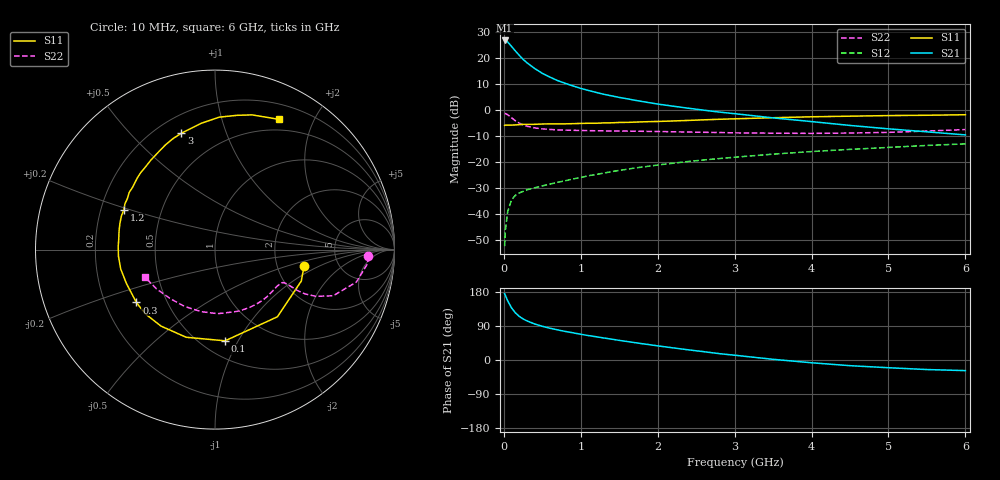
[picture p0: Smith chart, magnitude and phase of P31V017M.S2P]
! SIEMENS Small Signal Semiconductors
! BFP181
! Si NPN RF Bipolar Junction Transistor in SOT143
! VCE = 1 V  IC = 17 mA
! Common Emitter S-Parameters:  March  1996
# GHz  S  MA  R  50
!  f  S11  S21  S12  S22
! GHz  MAG  ANG  MAG  ANG  MAG  ANG  MAG  ANG
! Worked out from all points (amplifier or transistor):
!   36 points, 10 MHz to 6 GHz, reference 50 ohm
!   highest |S21| = 26.7 dB at 10 MHz (marker M1)
!   |S21| within 3 dB of that: start of sweep to 120.4 MHz
!   unconditionally stable (mu >= 1): start of sweep to 21.11 MHz; 260.1 MHz to end of sweep
!   at 250 MHz: K = 0.98, MSG = 25.4 dB, |S12| = -31.3 dB
!   at 1.4 GHz: K = 2.21, MAG = 8.4 dB, |S12| = -23.7 dB
!   at 6 GHz: K = 1.94, MAG = -3.9 dB, |S12| = -13.1 dB
!   S11 on the Smith chart (normalised r, x): 10 MHz: 2.85, -0.68; 100 MHz: 0.64, -0.88; 300 MHz: 0.33, -0.27; 1.2 GHz: 0.30, +0.19; 3 GHz: 0.30, +0.71; 6 GHz: 0.37, +1.54
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0.01  0.5045 -10.2  21.67 175.1  0.0024 74.9  0.8554 -2.5
0.02  0.5118 -20.0  21.6 170.4  0.0049 70.7  0.8523 -5.4
0.05  0.511 -47.1  20.22 156.2  0.0111 71.8  0.8085 -12.9
0.1  0.5113 -83.7  16.67 137.6  0.0186 55.5  0.7074 -21.3
0.15  0.5142 -108.2  13.61 124.5  0.0228 49.3  0.6191 -24.9
0.2  0.5217 -125.2  11.23 115.2  0.0253 45.8  0.5576 -26.2
0.25  0.5282 -137.5  9.399 108.3  0.0271 43.3  0.514 -26.4
0.3  0.5279 -146.1  8.083 103.3  0.0291 42.5  0.4857 -26.1
0.4  0.5285 -159.1  6.268 95.1  0.0318 43.0  0.4515 -25.6
0.5  0.5363 -168.4  5.053 89.0  0.0346 44.3  0.4323 -25.5
0.6  0.539 -175.9  4.274 83.8  0.0375 45.9  0.4209 -25.9
0.7  0.5396 178.3  3.661 79.4  0.0406 47.1  0.4134 -26.6
0.8  0.5398 173.2  3.241 75.3  0.0435 48.7  0.4093 -27.6
1.1  0.5541 160.2  2.369 64.4  0.0543 51.5  0.3995 -31.8
1.2  0.554 156.4  2.172 61.4  0.0575 51.4  0.3975 -33.5
1.7  0.5828 139.7  1.537 45.9  0.0764 51.9  0.3905 -42.8
2.2  0.6132 125.7  1.181 32.0  0.0945 49.9  0.3803 -53.6
3  0.6749 106.2  0.847 12.6  0.1232 44.5  0.3622 -73.3
3.5  0.7077 96.3  0.703 1.8  0.1411 40.7  0.3573 -87.6
4.5  0.7581 80.7  0.503 -15.0  0.1743 31.7  0.3593 -118.3
5.5  0.7901 69.1  0.379 -25.2  0.2077 22.7  0.3929 -146.3
6  0.8082 63.9  0.331 -28.0  0.2225 17.8  0.4192 -158.5
